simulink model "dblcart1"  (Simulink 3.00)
settings: Solver=ode23  SolverMode=SingleTasking  StartTime=0  StopTime=10000  MaxStep=0.1  RelTol=1e-3  AbsTol=1e-6
PreLoadFcn:
  | load dblcart1
undefined symbols (not defined in the file or in its folder): ae, be, ce, de, ka, m1, m2

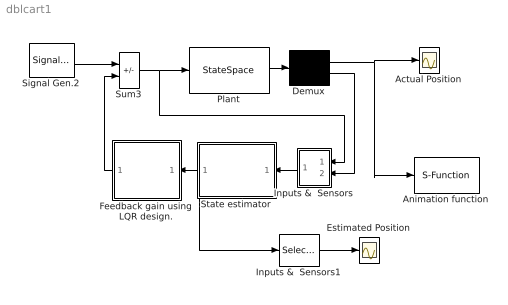
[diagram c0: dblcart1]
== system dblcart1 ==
  Actual Position : Scope
  Animation function : S-Function  FunctionName=crtanim2  Parameters=0.1  PortCounts=[]  SFunctionModules=''
  Demux : Demux  Outputs=[2,1]
  Estimated Position : Scope
  Feedback gain using LQR design. : Subsystem  Orientation=left  mask(Regulator){}
      mask help: Matrix Gain
      mask init:
      | k=@1;
  Inputs &  Sensors : Subsystem  Orientation=left
  Inputs &  Sensors1 : Selector  Elements=[1 3]  InputPortWidth=4
  Plant : StateSpace  A=[0 1 0 0; -ka/m1 0 ka/m1 0; 0 0 0 1;ka/m2 0 -ka/m2 0]  B=[0; 1; 0; 0]  C=[1 0 0 0;0 0 1 0;0 0 1 0]  D=zeros(3,1)  X0=0
  Signal Gen.2 : SignalGenerator  WaveForm=square  Amplitude=15  Frequency=0.300000  Units=rad/sec
  State estimator : Subsystem  Orientation=left
  Sum3 : Sum  Inputs=+-  SaturateOnIntegerOverflow=on
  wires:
  State estimator/1(Out1) -> Inputs &  Sensors1/1, Feedback gain using LQR design./1(In1)
  Inputs &  Sensors/1(Out1) -> State estimator/1(In1)
  Sum3/1 -> Inputs &  Sensors/1(In1), Plant/1
  Demux/1 -> Actual Position/1, Animation function/1
  Feedback gain using LQR design./1(Out1) -> Sum3/2
  Demux/2 -> Inputs &  Sensors/2(In2)
  Plant/1 -> Demux/1
  Signal Gen.2/1 -> Sum3/1
  Inputs &  Sensors1/1 -> Estimated Position/1

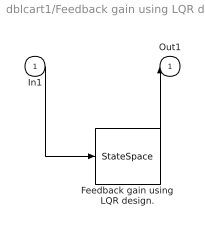
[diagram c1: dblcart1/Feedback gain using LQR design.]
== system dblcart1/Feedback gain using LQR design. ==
  In1 : Inport  Port=1  PortWidth=-1  SampleTime=-1  DataType=auto
  Feedback gain using LQR design. : StateSpace  A=[]  B=[]  C=[]  D=k  X0=0
  Out1 : Outport  Port=1  InitialOutput=0
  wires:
  In1/1 -> Feedback gain using LQR design./1
  Feedback gain using LQR design./1 -> Out1/1

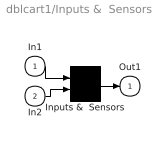
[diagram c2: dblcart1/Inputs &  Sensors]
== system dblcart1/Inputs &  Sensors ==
  In1 : Inport  Port=1  PortWidth=-1  SampleTime=-1  DataType=auto
  In2 : Inport  Port=2  PortWidth=-1  SampleTime=-1  DataType=auto
  Inputs &  Sensors : Mux  Inputs=2
  Out1 : Outport  Port=1  InitialOutput=0
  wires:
  In1/1 -> Inputs &  Sensors/1
  In2/1 -> Inputs &  Sensors/2
  Inputs &  Sensors/1 -> Out1/1

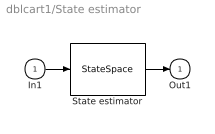
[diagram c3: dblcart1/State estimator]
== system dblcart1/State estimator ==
  In1 : Inport  Port=1  PortWidth=-1  SampleTime=-1  DataType=auto
  State estimator : StateSpace  A=ae  B=be  C=ce  D=de  X0=0
  Out1 : Outport  Port=1  InitialOutput=0
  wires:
  In1/1 -> State estimator/1
  State estimator/1 -> Out1/1
